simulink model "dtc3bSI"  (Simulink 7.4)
settings: Solver=ode45  StartTime=0.0  StopTime=.4  MaxStep=6e-7  RelTol=1e-3
InitFcn:
  | warning off; wmo=0.0%initial speed
  | fso=.996%initial stator flux
  | Vdc=700
  | wo=2*pi*60;
  | %
undefined symbols (not defined in the file or in its folder): a, wmo

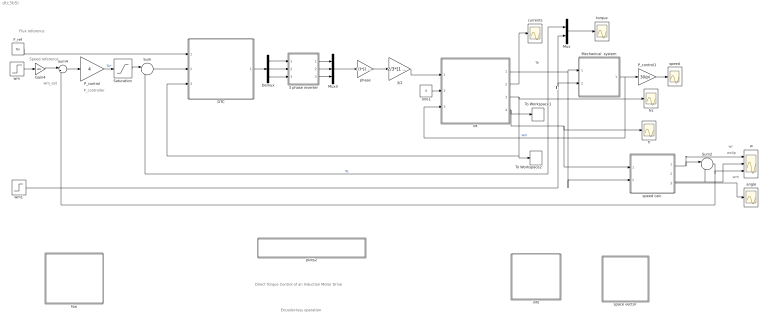
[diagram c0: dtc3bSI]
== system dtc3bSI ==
  note: Direct Torque Control of an Induction Motor Drive
  note: Flux reference
  note: Speed reference
  note: Te
  note: Tl
  note: P_controller
  note: Encoder-less operation
  note: wr
  note: wslip
  note: wm
  note: wm_est
  3 phase inverter : Subsystem
  3/2 : Gain  Gain=2/3*[1 -0.5 -0.5;0 sqrt(3)/2 -sqrt(3)/2]  Multiplication=Matrix(K*u)  ParameterDataType=sfix(16)  ParameterScaling=2^0  OutDataType=sfix(16)  OutScaling=2^0
  DTC : Subsystem
  Demux : Demux  Outputs=3
  F_ref : Constant  Value=fso  OutDataType=sfix(16)  OutScaling=2^0
  Gain4 : Gain  Gain=wo  ParameterDataType=sfix(16)  ParameterScaling=2^0  OutDataType=sfix(16)  OutScaling=2^0
  IM : Subsystem  mask{Rs=1.77, Rr=1.34, Lsl=13.93e-3, Lrl=12.12e-3, Lm=369e-3, p=4}
      mask prompts: Rs "Stator resistance [Ohm]"; Rr "Rotor resistance [Ohm]"; Lsl "Stator leakage inductance [H]"; Lrl "Rotor leakage inductance [H]"; Lm "Magnetizing inductance [H]"; p "Number of poles"
  Mechanical  system : Subsystem  mask{J=0.025, Bm=1e-5}
      mask prompts: J "Moment of inertia [Kg.m^2]"; Bm "Torque-speed coefficient"
  Mux : Mux  Inputs=2
  Mux3 : Mux  Inputs=3
  P_control : Gain  Gain=4  ParameterDataType=sfix(16)  ParameterScaling=2^0  OutDataType=sfix(16)  OutScaling=2^0
  P_control1 : Gain  Gain=30/pi  ParameterDataType=sfix(16)  ParameterScaling=2^0  OutDataType=sfix(16)  OutScaling=2^0
  Saturation : Saturate  UpperLimit=30  LowerLimit=-30
  Sum : Sum  Inputs=|+-  OutDataType=sfix(16)  OutScaling=2^0
  Sum2 : Sum  Inputs=|+-  OutDataType=sfix(16)  OutScaling=2^0
  Sum4 : Sum  Inputs=|+-  OutDataType=sfix(16)  OutScaling=2^0
  To Workspace1 : ToWorkspace  VariableName=fr  SampleTime=-1  SaveFormat=Array
  To Workspace2 : ToWorkspace  VariableName=fs  SampleTime=-1  SaveFormat=Array
  angle : Scope
  currents : Scope
  fr : Scope
  frs : Scope
  fsw : Subsystem
  info : Subsystem
  one1 : Constant  Value=0  OutDataType=sfix(16)  OutScaling=2^0
  phase : Gain  Gain=1/3*[2 -1 -1;-1 2 -1;-1 -1 2]  Multiplication=Matrix(K*u)  ParameterDataType=sfix(16)  ParameterScaling=2^0  OutDataType=sfix(16)  OutScaling=2^0
  plots2 : Subsystem
  space vector : Subsystem
  speed : Scope
  speed calc : Subsystem
  torque : Scope
  w : Scope  NumInputPorts=3
  wm : Step  Time=.05  Before=wmo  After=.8  SampleTime=0
  wm1 : Step  Time=.3  After=12  SampleTime=0
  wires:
  F_ref/1 -> DTC/1(f_ref)
  3/2/1 -> IM/1(vs)
  IM/3(fs) -> To Workspace2/1, DTC/3(fs), frs/1
  one1/1 -> IM/2(wk)
  IM/1(Te) -> Mux/1, Mechanical  system/1(Te), speed calc/2(Te), Sum/2  "Te"
  Mechanical  system/1(wm) -> IM/3(wmec), P_control1/1  "wm"
  IM/2(is) -> currents/1
  wm/1 -> Gain4/1
  Sum/1 -> DTC/2(T_er)
  Mux/1 -> torque/1
  Sum4/1 -> P_control/1
  P_control/1 -> Saturation/1  "Te*"
  IM/4(fr) -> To Workspace1/1, fr/1, speed calc/1(fr)
  wm1/1 -> Mux/2, Mechanical  system/2(Tl)
  Saturation/1 -> Sum/1
  speed calc/1(wr) -> Sum2/1, w/1
  speed calc/2(wslip) -> Sum2/2, w/2
  Sum2/1 -> w/3, Sum4/2
  Mux3/1 -> phase/1
  Demux/1 -> 3 phase inverter/1(sa)
  Demux/2 -> 3 phase inverter/2(sb)
  Demux/3 -> 3 phase inverter/3(sc)
  3 phase inverter/1(va) -> Mux3/1
  3 phase inverter/2(vb) -> Mux3/2
  3 phase inverter/3(vc) -> Mux3/3
  DTC/1(s3) -> Demux/1
  phase/1 -> 3/2/1
  Gain4/1 -> Sum4/1
  P_control1/1 -> speed/1
  speed calc/3(an) -> angle/1

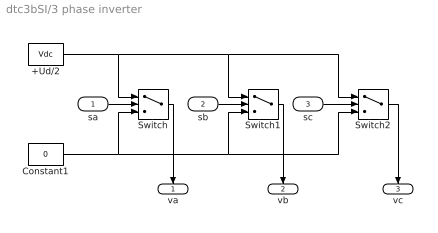
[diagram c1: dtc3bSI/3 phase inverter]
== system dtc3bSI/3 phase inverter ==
  sa : Inport  OutDataType=sfix(16)  OutScaling=2^0
  sb : Inport  Port=2  OutDataType=sfix(16)  OutScaling=2^0
  sc : Inport  Port=3  OutDataType=sfix(16)  OutScaling=2^0
  +Ud/2 : Constant  Value=Vdc  OutDataType=sfix(16)  OutScaling=2^0
  Constant1 : Constant  Value=0  OutDataType=sfix(16)  OutScaling=2^0
  Switch : Switch  Threshold=0.5
  Switch1 : Switch  Threshold=0.5
  Switch2 : Switch  Threshold=0.5
  va : Outport  InitialOutput=0
  vb : Outport  Port=2  InitialOutput=0
  vc : Outport  Port=3  InitialOutput=0
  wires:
  Switch1/1 -> vb/1
  Switch2/1 -> vc/1
  sc/1 -> Switch2/2
  sb/1 -> Switch1/2
  Switch/1 -> va/1
  sa/1 -> Switch/2
  Constant1/1 -> Switch2/3, Switch1/3, Switch/3
  +Ud/2/1 -> Switch2/1, Switch1/1, Switch/1

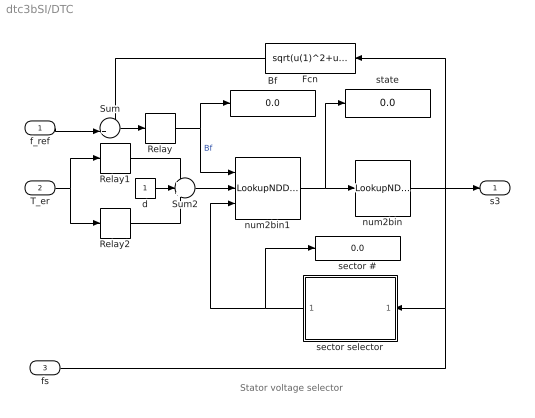
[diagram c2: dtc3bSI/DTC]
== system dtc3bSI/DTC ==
  note: Stator voltage selector
  f_ref : Inport  OutDataType=sfix(16)  OutScaling=2^0
  T_er : Inport  Port=2  OutDataType=sfix(16)  OutScaling=2^0
  fs : Inport  Port=3  OutDataType=sfix(16)  OutScaling=2^0
  Bf : Display
  Fcn : Fcn  Expr=sqrt(u(1)^2+u(2)^2)
  Relay : Relay  OnSwitchValue=.02  OffSwitchValue=-.02  OutDataType=sfix(16)  OutScaling=2^0
  Relay1 : Relay  OnSwitchValue=.2  OffSwitchValue=0  OutDataType=sfix(16)  OutScaling=2^0  ZeroCross=off
  Relay2 : Relay  OnSwitchValue=0  OffSwitchValue=-.2  OnOutputValue=0  OffOutputValue=-1  OutDataType=sfix(16)  OutScaling=2^0  ZeroCross=off
  Sum : Sum  Inputs=-+|  OutDataType=sfix(16)  OutScaling=2^0
  Sum2 : Sum  Inputs=+++  OutDataType=sfix(16)  OutScaling=2^0
  d : Constant  OutDataType=sfix(16)  OutScaling=2^0
  num2bin : LookupNDDirect  InputsSelectThisObjectFromTable=Column  Table=[0 0 0;1 0 0;0 1 0;1 1 0;0 0 1;1 0 1;0 1 1;1 1 1]'  ActionForOutOfRangeInput=Error
  num2bin1 : LookupNDDirect  NumberOfTableDimensions=3  Table=a  ActionForOutOfRangeInput=Error
  sector # : Display
  sector selector : Subsystem
  state : Display
  s3 : Outport
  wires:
  num2bin1/1 -> state/1, num2bin/1
  Sum/1 -> Relay/1
  Relay/1 -> Bf/1, num2bin1/1  "Bf"
  Fcn/1 -> Sum/1
  Sum2/1 -> num2bin1/2
  Relay1/1 -> Sum2/1
  Relay2/1 -> Sum2/3
  d/1 -> Sum2/2
  T_er/1 -> Relay2/1, Relay1/1
  f_ref/1 -> Sum/2
  num2bin/1 -> s3/1
  fs/1 -> Fcn/1, sector selector/1(fs)
  sector selector/1(sector) -> num2bin1/3, sector #/1

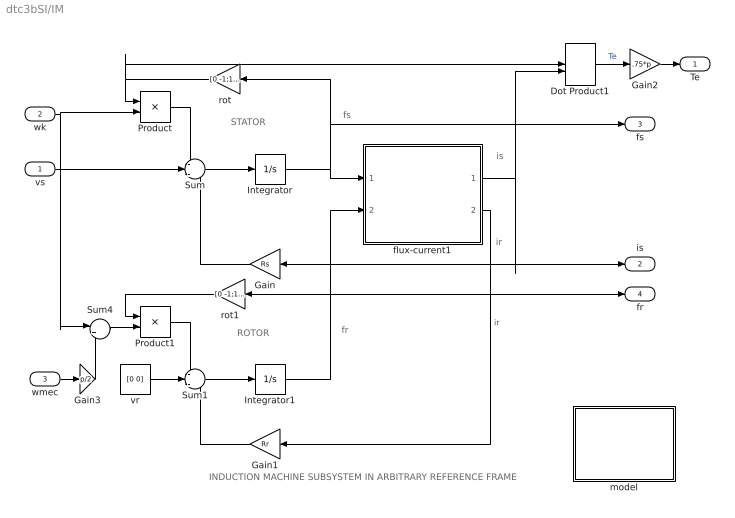
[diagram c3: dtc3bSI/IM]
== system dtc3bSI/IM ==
  note: ROTOR
  note: STATOR
  note: fs
  note: fr
  note: is
  note: INDUCTION MACHINE SUBSYSTEM IN ARBITRARY REFERENCE FRAME
  note: ir
  vs : Inport  OutDataType=sfix(16)  OutScaling=2^0
  wk : Inport  Port=2  OutDataType=sfix(16)  OutScaling=2^0
  wmec : Inport  Port=3  OutDataType=sfix(16)  OutScaling=2^0
  Dot Product1 : DotProduct  OutDataType=fixdt(1, 16)  OutScaling=2^-10
  Gain : Gain  Gain=Rs  ParameterDataType=sfix(16)  ParameterScaling=2^0  OutDataType=sfix(16)  OutScaling=2^0
  Gain1 : Gain  Gain=Rr  ParameterDataType=sfix(16)  ParameterScaling=2^0  OutDataType=sfix(16)  OutScaling=2^0
  Gain2 : Gain  Gain=.75*p  ParameterDataType=sfix(16)  ParameterScaling=2^0  OutDataType=sfix(16)  OutScaling=2^0
  Gain3 : Gain  Gain=p/2  ParameterDataType=sfix(16)  ParameterScaling=2^0  OutDataType=sfix(16)  OutScaling=2^0
  Integrator : Integrator  InitialCondition=[fso 0]
  Integrator1 : Integrator  InitialCondition=[fso 0]
  Product : Product  OutDataType=sfix(16)  OutScaling=2^0
  Product1 : Product  OutDataType=sfix(16)  OutScaling=2^0
  Sum : Sum  Inputs=-+-  OutDataType=sfix(16)  OutScaling=2^0
  Sum1 : Sum  Inputs=-+-  OutDataType=sfix(16)  OutScaling=2^0
  Sum4 : Sum  Inputs=|+-  OutDataType=sfix(16)  OutScaling=2^0
  flux-current1 : Subsystem
  model : Subsystem
  rot : Gain  Gain=[0 -1;1 0]  Multiplication=Matrix(K*u)  ParameterDataType=sfix(16)  ParameterScaling=2^0  OutDataType=sfix(16)  OutScaling=2^0
  rot1 : Gain  Gain=[0 -1;1 0]  Multiplication=Matrix(K*u)  ParameterDataType=sfix(16)  ParameterScaling=2^0  OutDataType=sfix(16)  OutScaling=2^0
  vr : Constant  Value=[0 0]  OutDataType=sfix(16)  OutScaling=2^0
  Te : Outport
  is : Outport  Port=2
  fs : Outport  Port=3
  fr : Outport  Port=4
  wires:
  Gain/1 -> Sum/3
  vr/1 -> Sum1/2
  Gain1/1 -> Sum1/3
  flux-current1/2(ir) -> Gain1/1  "ir"
  Integrator/1 -> flux-current1/1(fs), rot/1, fs/1
  Integrator1/1 -> flux-current1/2(fr), rot1/1, fr/1
  Product1/1 -> Sum1/1
  rot1/1 -> Product1/1
  Product/1 -> Sum/1
  rot/1 -> Product/1, Dot Product1/1
  Sum4/1 -> Product1/2
  Sum/1 -> Integrator/1
  Sum1/1 -> Integrator1/1
  flux-current1/1(is) -> Gain/1, is/1, Dot Product1/2
  Dot Product1/1 -> Gain2/1  "Te"
  vs/1 -> Sum/2
  wk/1 -> Product/2, Sum4/1
  wmec/1 -> Gain3/1
  Gain2/1 -> Te/1
  Gain3/1 -> Sum4/2

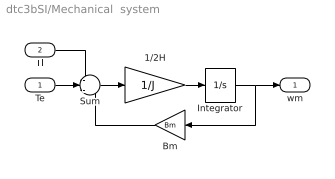
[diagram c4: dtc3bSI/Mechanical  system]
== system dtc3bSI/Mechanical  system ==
  Te : Inport  OutDataType=sfix(16)  OutScaling=2^0
  Tl : Inport  Port=2  OutDataType=sfix(16)  OutScaling=2^0
  1/2H : Gain  Gain=1/J  ParameterDataType=sfix(16)  ParameterScaling=2^0  OutDataType=sfix(16)  OutScaling=2^0
  Bm : Gain  Gain=Bm  ParameterDataType=sfix(16)  ParameterScaling=2^0  OutDataType=sfix(16)  OutScaling=2^0
  Integrator : Integrator  InitialCondition=wmo
  Sum : Sum  Inputs=-+-  OutDataType=sfix(16)  OutScaling=2^0
  wm : Outport
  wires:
  Tl/1 -> Sum/1
  Te/1 -> Sum/2
  Integrator/1 -> wm/1, Bm/1
  Bm/1 -> Sum/3
  Sum/1 -> 1/2H/1
  1/2H/1 -> Integrator/1

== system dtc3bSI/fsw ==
  note: Script files
  note: This collection of demonstrations is designed to illustrate the use of MATLAB for the simulation of the steady-state characteristics of ac machines under balanced and unbalanced conditions of operation.

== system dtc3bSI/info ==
  note: Direct torque control of an induction motordrive
  note: The induction motor operates initially at no load at a speed and a stator flux level specified in a callback of the model properties. The mechanical load torque is initially set at Tl = 0 and the electromagnetic torque Te is set to zero by having stator and rotor space vectors colinear (check the IC's of the flux integrators). Before running, double click the Switching Table block.

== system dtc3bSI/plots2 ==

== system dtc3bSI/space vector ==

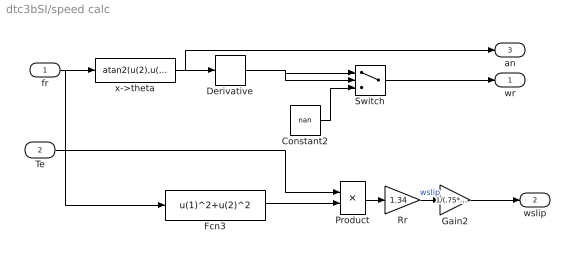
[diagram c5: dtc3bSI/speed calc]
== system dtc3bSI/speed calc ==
  fr : Inport  OutDataType=sfix(16)  OutScaling=2^0
  Te : Inport  Port=2  OutDataType=sfix(16)  OutScaling=2^0
  Constant2 : Constant  Value=nan  OutDataType=sfix(16)  OutScaling=2^0
  Derivative : Derivative
  Fcn3 : Fcn  Expr=u(1)^2+u(2)^2
  Gain2 : Gain  Gain=1/(.75*4)  ParameterDataType=sfix(16)  ParameterScaling=2^0  OutDataType=sfix(16)  OutScaling=2^0
  Product : Product  Inputs=*/  OutDataType=sfix(16)  OutScaling=2^0
  Rr : Gain  Gain=1.34  ParameterDataType=sfix(16)  ParameterScaling=2^0  OutDataType=sfix(16)  OutScaling=2^0
  Switch : Switch  ZeroCross=off
  x->theta : Fcn  Expr=atan2(u(2),u(1))
  wr : Outport
  wslip : Outport  Port=2
  an : Outport  Port=3
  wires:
  Switch/1 -> wr/1
  Constant2/1 -> Switch/3
  Derivative/1 -> Switch/1, Switch/2
  fr/1 -> x->theta/1, Fcn3/1
  x->theta/1 -> Derivative/1, an/1
  Fcn3/1 -> Product/2
  Product/1 -> Rr/1
  Te/1 -> Product/1
  Rr/1 -> Gain2/1  "wslip"
  Gain2/1 -> wslip/1

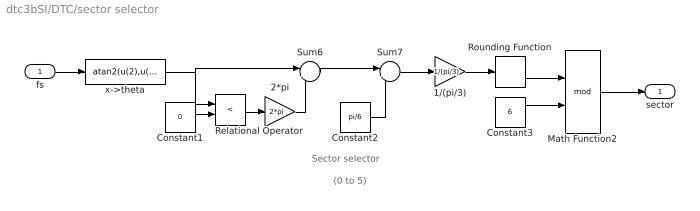
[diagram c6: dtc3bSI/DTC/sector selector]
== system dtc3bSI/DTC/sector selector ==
  note: Sector selector
  note: (0 to 5)
  fs : Inport  OutDataType=sfix(16)  OutScaling=2^0
  1/(pi/3) : Gain  Gain=1/(pi/3)  ParameterDataType=sfix(16)  ParameterScaling=2^0  OutDataType=sfix(16)  OutScaling=2^0
  2*pi : Gain  Gain=2*pi  ParameterDataType=sfix(16)  ParameterScaling=2^0  OutDataType=sfix(16)  OutScaling=2^0
  Constant1 : Constant  Value=0  OutDataType=sfix(16)  OutScaling=2^0
  Constant2 : Constant  Value=pi/6  OutDataType=sfix(16)  OutScaling=2^0
  Constant3 : Constant  Value=6  OutDataType=sfix(16)  OutScaling=2^0
  Math Function2 : Math  Operator=mod
  Relational Operator : RelationalOperator  Operator=<
  Rounding Function : Rounding
  Sum6 : Sum  Inputs=|++  OutDataType=sfix(16)  OutScaling=2^0
  Sum7 : Sum  Inputs=|++  OutDataType=sfix(16)  OutScaling=2^0
  x->theta : Fcn  Expr=atan2(u(2),u(1))
  sector : Outport
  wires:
  Constant1/1 -> Relational Operator/2
  Relational Operator/1 -> 2*pi/1
  2*pi/1 -> Sum6/2
  Sum6/1 -> Sum7/1
  Constant2/1 -> Sum7/2
  Sum7/1 -> 1/(pi/3)/1
  1/(pi/3)/1 -> Rounding Function/1
  Rounding Function/1 -> Math Function2/1
  Constant3/1 -> Math Function2/2
  fs/1 -> x->theta/1
  Math Function2/1 -> sector/1
  x->theta/1 -> Relational Operator/1, Sum6/1

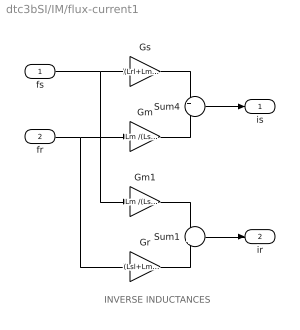
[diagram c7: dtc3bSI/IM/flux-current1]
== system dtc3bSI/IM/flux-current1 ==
  note: INVERSE INDUCTANCES
  fs : Inport  OutDataType=sfix(16)  OutScaling=2^0
  fr : Inport  Port=2  OutDataType=sfix(16)  OutScaling=2^0
  Gm : Gain  Gain=Lm /(Lsl*Lrl+Lsl*Lm+Lrl*Lm)  ParameterDataType=sfix(16)  ParameterScaling=2^0  OutDataType=sfix(16)  OutScaling=2^0
  Gm1 : Gain  Gain=Lm /(Lsl*Lrl+Lsl*Lm+Lrl*Lm)  ParameterDataType=sfix(16)  ParameterScaling=2^0  OutDataType=sfix(16)  OutScaling=2^0
  Gr : Gain  Gain=(Lsl+Lm )/(Lsl*Lrl+Lsl*Lm+Lrl*Lm)  ParameterDataType=sfix(16)  ParameterScaling=2^0  OutDataType=sfix(16)  OutScaling=2^0
  Gs : Gain  Gain=(Lrl+Lm) /(Lsl*Lrl+Lsl*Lm+Lrl*Lm)  ParameterDataType=sfix(16)  ParameterScaling=2^0  OutDataType=sfix(16)  OutScaling=2^0
  Sum1 : Sum  Inputs=-+  OutDataType=sfix(16)  OutScaling=2^0
  Sum4 : Sum  Inputs=+-  OutDataType=sfix(16)  OutScaling=2^0
  is : Outport
  ir : Outport  Port=2
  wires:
  fs/1 -> Gs/1, Gm1/1
  Gs/1 -> Sum4/1
  fr/1 -> Gm/1, Gr/1
  Gm/1 -> Sum4/2
  Sum4/1 -> is/1
  Gm1/1 -> Sum1/1
  Gr/1 -> Sum1/2
  Sum1/1 -> ir/1

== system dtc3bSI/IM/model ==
  note: Mathematical model of the induction machine. State vector formulation in an arbitrary dq common reference frame. Per unit description.
  note: Electrical system equations: vs = Rs is + 1/wo (dfs/dt) + wk M(pi/2) fs vr = Rr ir + 1/wo (dfr/dt) + (wk - wm) M(pi/2) fr where the variables i, v, and f are 2-dimensional space vectors; for instance is = [ids iqs] and so forth, wk is the speed of the reference frame, wm the rotor speed, and M(pi/2)represents a 90o space rotator namely M(pi/2) = [0 -1;1 0] The flux linkage current relations are: fds = Ls ids + Lm idr fdr = Lm ids + Lr idr (D_axis) Ls =Lm +Lsl ; Lr = Lm +Lrl fqs = Ls iqs + Lm iqr fqr = Lm iqs + Lr iqr (Q_axis) Mechanical system equations: Te = 2H (dwm/dt ) + Bm wm + Tl where Te = fs (cross) is = M(pi/2) fs (dot) is = fds iqs - fqs ids = fs x is = M(pi/2) fs . is = ir x fr = Lm (ir x is) = Lm/Lr (fr x is) = 1/Lm' (fr x fs) Lm' =Lm c/(1-c) c = 1 - Lm^2/(Ls Lr)
